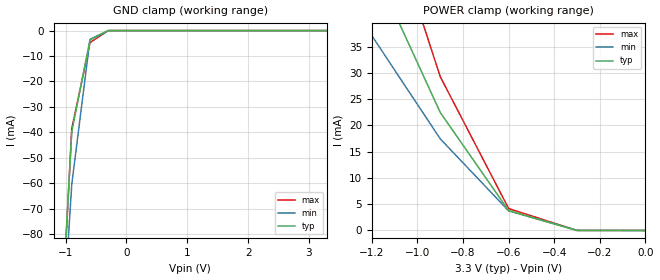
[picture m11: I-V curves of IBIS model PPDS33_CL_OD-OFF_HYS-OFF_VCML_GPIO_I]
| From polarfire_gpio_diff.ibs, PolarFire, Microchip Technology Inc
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|   Model PPDS33_CL_OD-OFF_HYS-OFF_VCML_GPIO_I
[Model]   PPDS33_CL_OD-OFF_HYS-OFF_VCML_GPIO_I
Model_type   Input
Vinl =   0.275
Vinh =   0.525
|   typ   min   max
C_comp_pullup   2.605e-12   2.605e-12   2.76e-12
C_comp_pulldown  2.605e-12   2.605e-12   2.76e-12
[Temperature Range]  25C   100C   -40C
[Voltage Range]  3.3   3.15   3.45
[GND_clamp]
|Voltage   I(typ)   I(min)   I(max)
-1.8V     -463.2mA   -408.7mA   -523.6mA
-1.2V     -171.2mA   -174.2mA   -177.2mA
-900mV    -39.7mA    -60.43mA   -38.53mA
-600mV    -3.657mA   -3.442mA   -4.73mA
-300mV    -2.517uA   -9.735uA   -1.044uA
3.3V      1.341uA    1.798uA    1.108uA
[POWER_clamp]
|Voltage   I(typ)   I(min)   I(max)
-3.3V     410.6mA    333.1mA    508mA
-3V       342.4mA    274.4mA    434mA
-2.7V     283.6mA    221.8mA    365.8mA
-2.4V     228.4mA    175.3mA    298.9mA
-2.1V     176.1mA    133mA      234.8mA
-1.8V     128.3mA    95.36mA    175.2mA
-1.5V     86.43mA    63.24mA    119.9mA
-1.2V     50.84mA    37.1mA     69.35mA
-900mV    22.47mA    17.45mA    29.29mA
-600mV    3.773mA    3.733mA    4.175mA
-300mV    6.226uA    20.37uA    3.158uA
0V        0A         0A         0A
